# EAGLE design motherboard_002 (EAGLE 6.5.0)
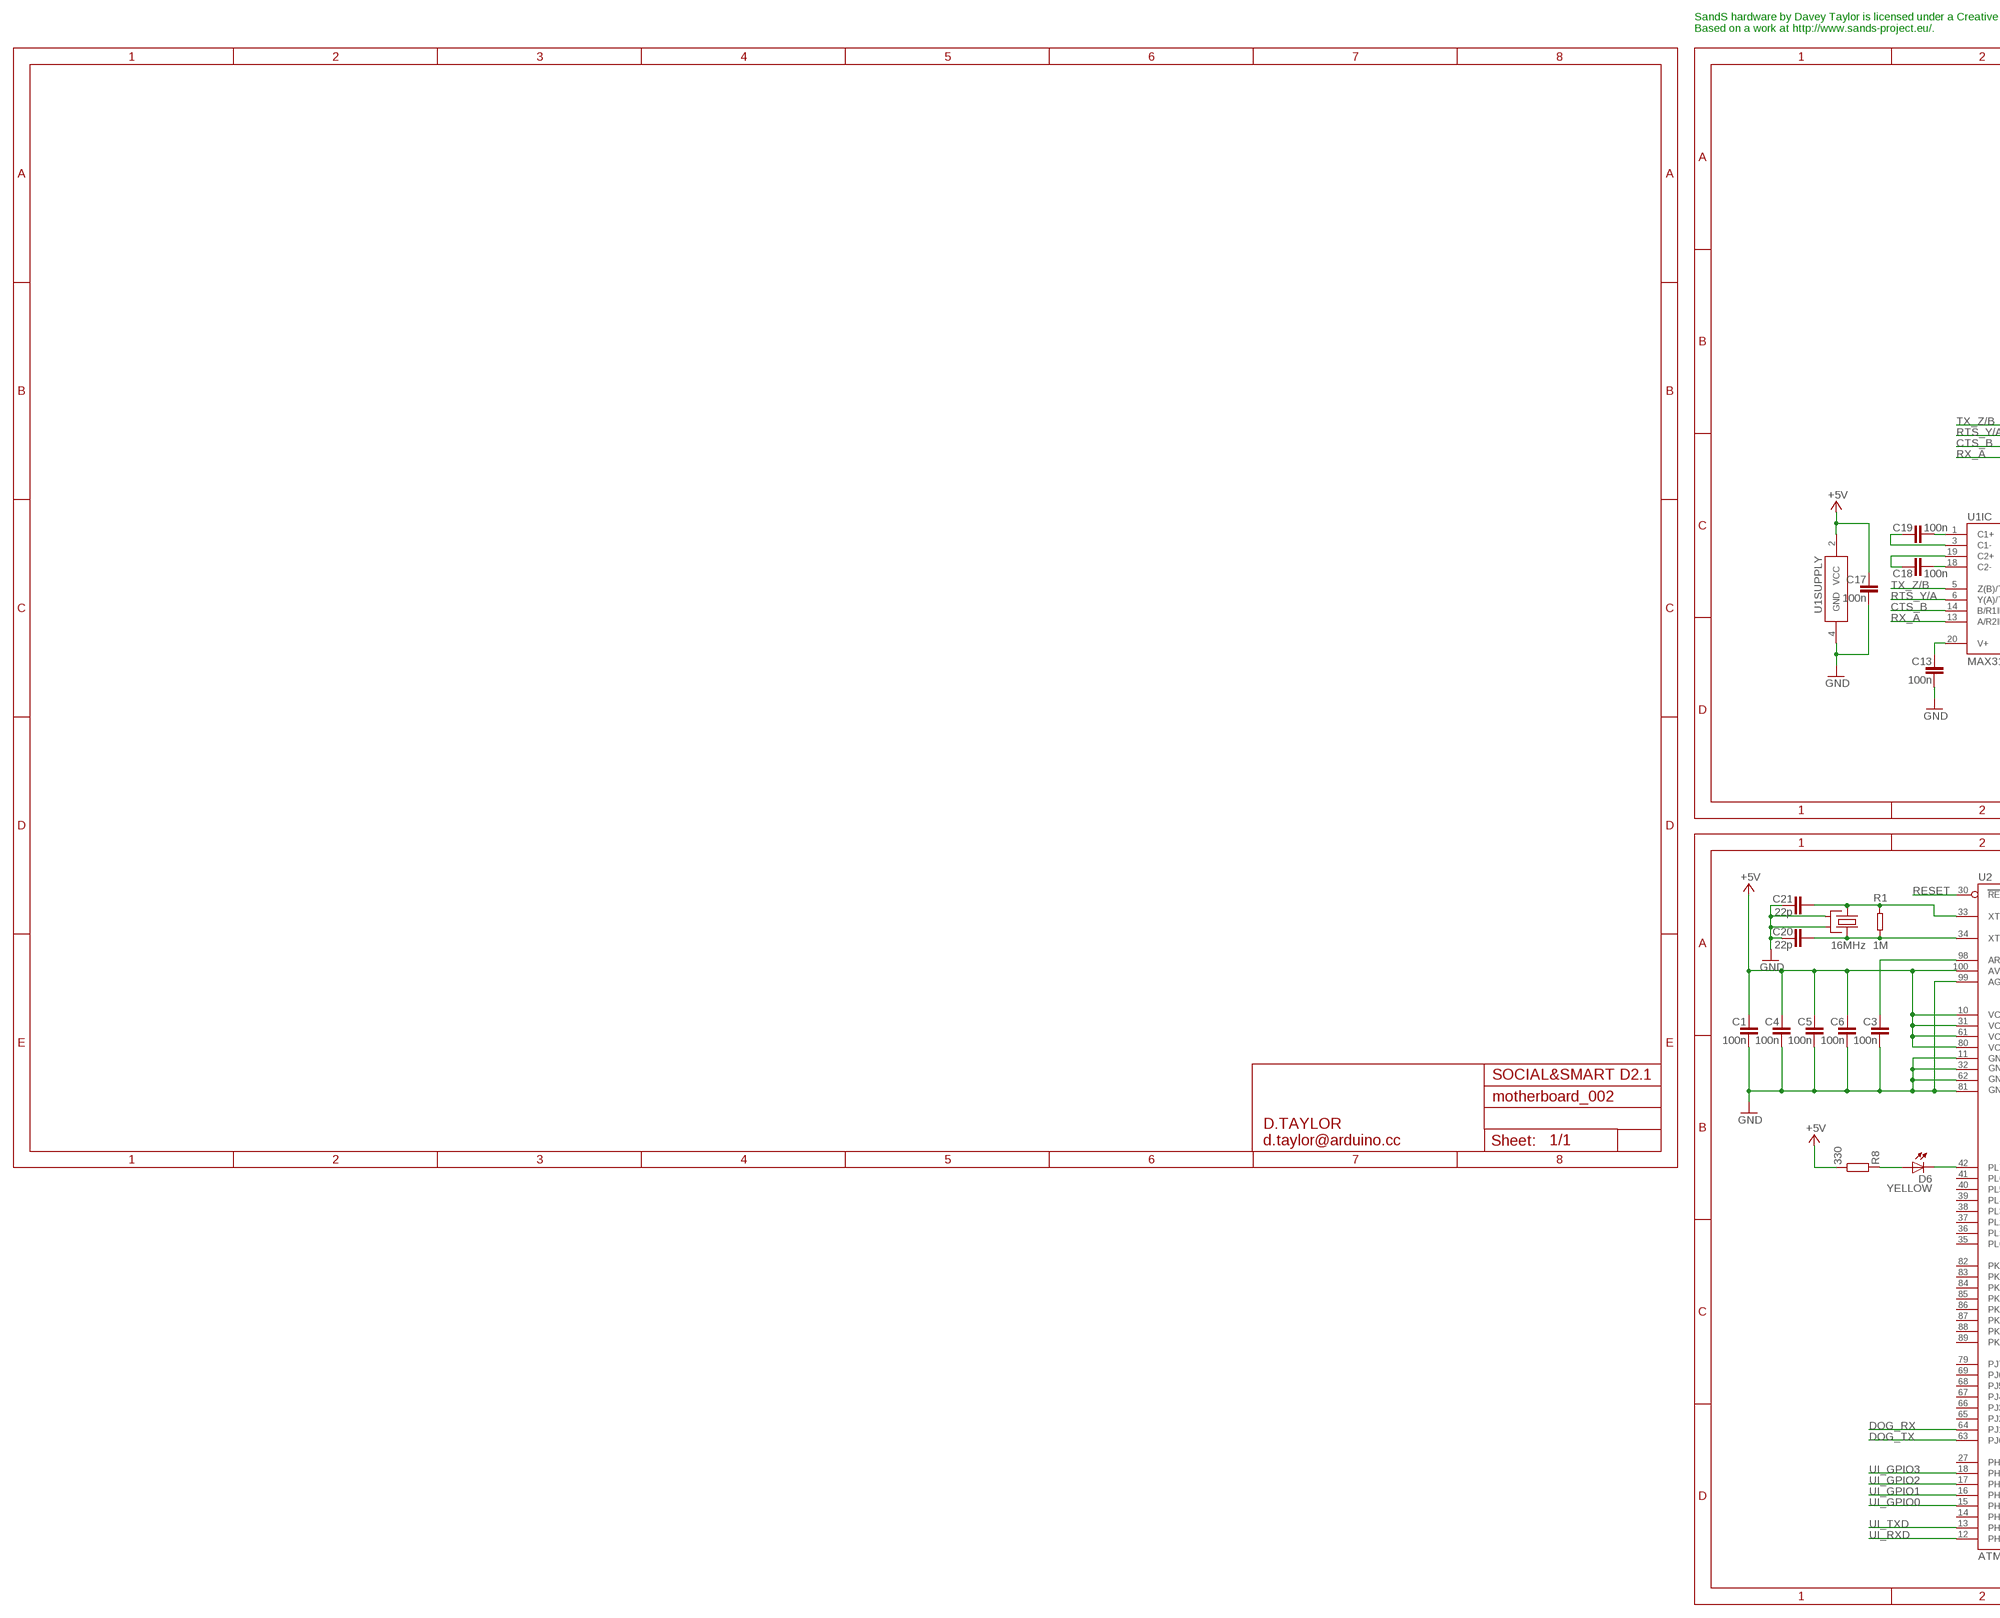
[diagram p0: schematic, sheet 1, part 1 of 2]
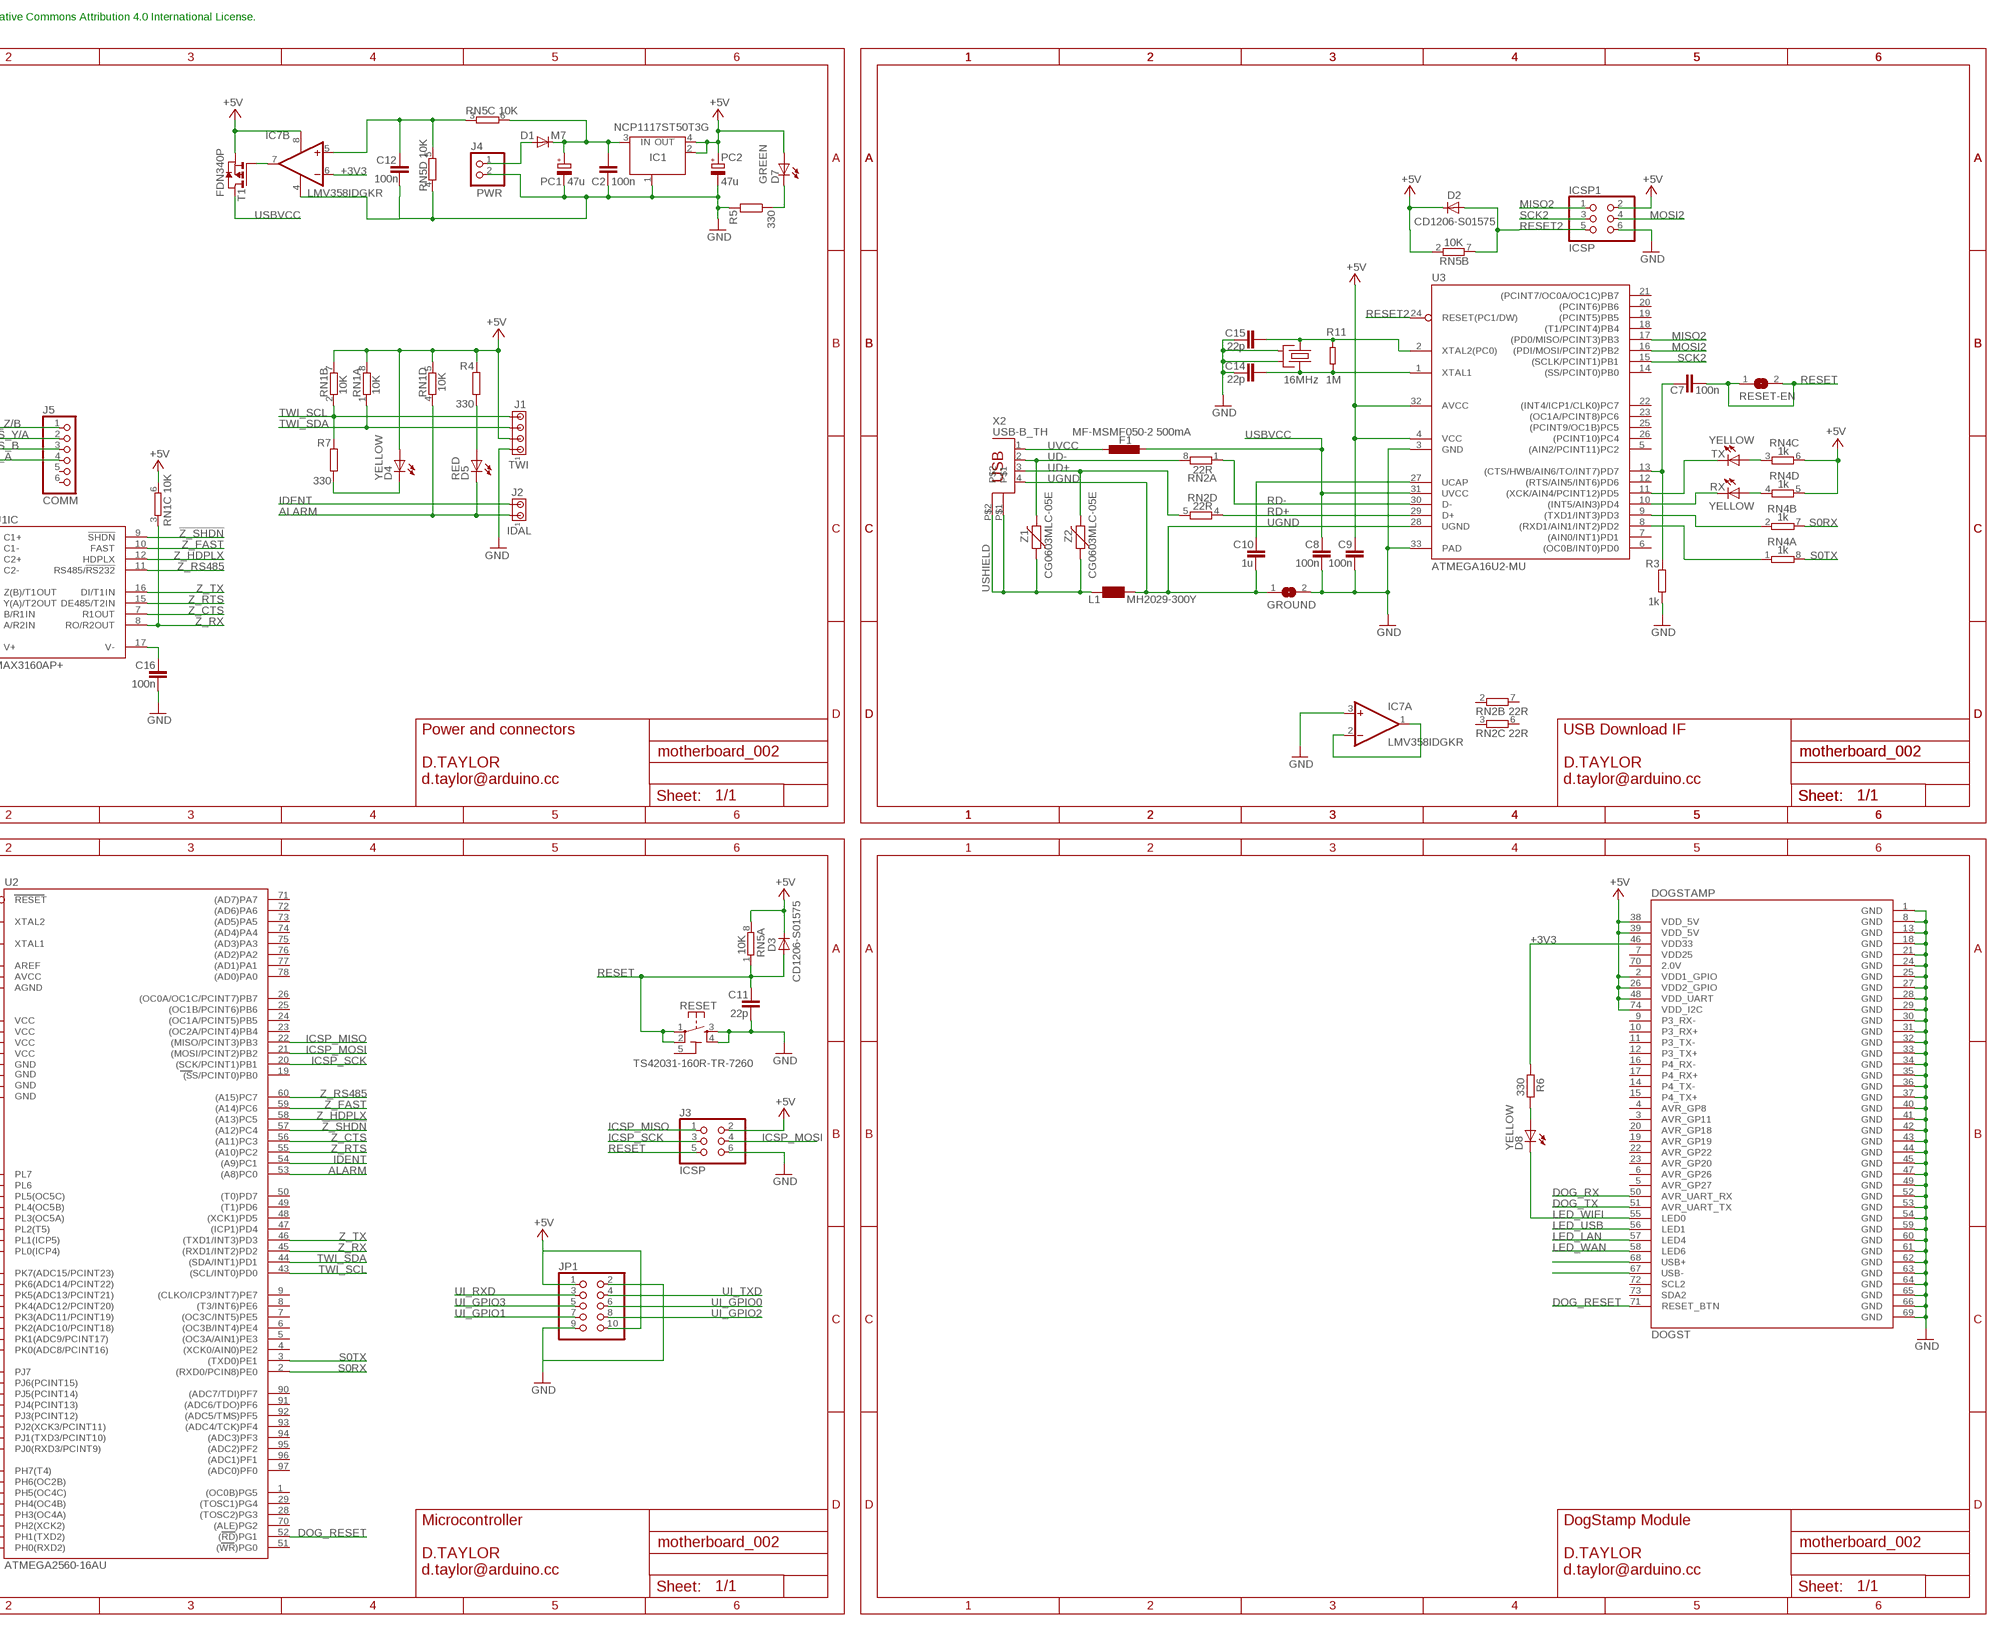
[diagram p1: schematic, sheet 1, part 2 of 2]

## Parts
C1  100n  C-EU0603-RND  [C0603-ROUND]
C2  100n  C-EU0603-RND  [C0603-ROUND]
C3  100n  C-EU0603-RND  [C0603-ROUND]
C4  100n  C-EU0603-RND  [C0603-ROUND]
C5  100n  C-EU0603-RND  [C0603-ROUND]
C6  100n  C-EU0603-RND  [C0603-ROUND]
C7  100n  C-EU0603-RND  [C0603-ROUND]
C8  100n  C-EU0603-RND  [C0603-ROUND]
C9  100n  C-EU0603-RND  [C0603-ROUND]
C10  1u  C-EU0603-RND  [C0603-ROUND]
C11  22p  C-EU0603-RND  [C0603-ROUND]
C12  100n  C-EU0603-RND  [C0603-ROUND]
C13  100n  C-EU0603-RND  [C0603-ROUND]
C14  22p  C-EU0603-RND  [C0603-ROUND]
C15  22p  C-EU0603-RND  [C0603-ROUND]
C16  100n  C-EU0603-RND  [C0603-ROUND]
C17  100n  C-EU0603-RND  [C0603-ROUND]
C18  100n  C-EU0603-RND  [C0603-ROUND]
C19  100n  C-EU0603-RND  [C0603-ROUND]
C20  22p  C-EU0603-RND  [C0603-ROUND]
C21  22p  C-EU0603-RND  [C0603-ROUND]
D1  M7  DIODE-SMB  [SMB]
D2  CD1206-S01575  DIODE-MINIMELF  [MINIMELF]
D3  CD1206-S01575  DIODE-MINIMELF  [MINIMELF]
D4  YELLOW  LEDCHIP-LED0805  [CHIP-LED0805]
D5  RED  LEDCHIP-LED0805  [CHIP-LED0805]
D6  YELLOW  LEDCHIP-LED0805  [CHIP-LED0805]
D7  GREEN  LEDCHIP-LED0805  [CHIP-LED0805]
D8  YELLOW  LEDCHIP-LED0805  [CHIP-LED0805]
DOGSTAMP  DOGST  [DOGST]
F1  MF-MSMF050-2 500mA  L-EUL1812  [L1812]
GROUND  SJ  [SJ]
IC1  NCP1117ST50T3G  MC33269ST-3.3T3  [SOT223]
IC7  LMV358IDGKR  LMV358MMX  [MSOP08]
ICSP1  ICSP  PINHD-2X3  [2X03]
J1  TWI  MTA04-100  [10X04MTA]
J2  IDAL  MTA02-100  [10X02MTA]
J3  ICSP  PINHD-2X3  [2X03]
J4  PWR  MKDS_1,5/2-5,08  [MKDS1,5/2-5,08]
J5  COMM  PINHD-1X6  [1X06]
JP1  PINHD-2X5  [2X05]
L1  MH2029-300Y  WE-CBF_0805  [0805]
PC1  47u  CPOL-EUD  [PANASONIC_D]
PC2  47u  CPOL-EUD  [PANASONIC_D]
R1  1M  R-EU_0603-RND  [R0603-ROUND]
R3  1k  R-EU_R0603  [R0603-ROUND]
R4  330  R-EU_R0603  [R0603-ROUND]
R5  330  R-EU_R0603  [R0603-ROUND]
R6  330  R-EU_R0603  [R0603-ROUND]
R7  330  R-EU_R0603  [R0603-ROUND]
R8  330  R-EU_R0603  [R0603-ROUND]
R11  1M  R-EU_0603-RND  [R0603-ROUND]
RESET  TS42031-160R-TR-7260  TS42  [TS42]
RESET-EN  SJ  [SJ]
RN1  10K  4R-NCAT16  [CAT16]
RN2  22R  4R-NCAY16  [CAY16]
RN4  1k  4R-NCAY16  [CAY16]
RN5  10K  4R-NCAT16  [CAT16]
RX  YELLOW  LEDCHIP-LED0805  [CHIP-LED0805]
T1  FDN340P  PMOSSOT23  [SOT-23]
TX  YELLOW  LEDCHIP-LED0805  [CHIP-LED0805]
U1  MAX3160AP+  [SSOP20]
U2  ATMEGA2560-16AU  ATMEGA25602560-16AU  [TQFP100]
U3  ATMEGA16U2-MU  [MLF32]
X1  16MHz  CRYSTAL2-KX7  [XTAL-3.2-2.5]
X2  USB-B_TH  PN61729  [PN61729]
X3  16MHz  CRYSTAL2-KX7  [XTAL-3.2-2.5]
Z1  CG0603MLC-05E  VARISTORCN0603  [CT/CN0603]
Z2  CG0603MLC-05E  VARISTORCN0603  [CT/CN0603]

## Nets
!Z_SHDN!: U1.9(IC:!SHDN!) U2.57((A12)PC4)
+3V3 [power]: DOGSTAMP.46(VDD33) IC7.6(B:-IN) R6.2
+5V: C1.1 C4.1 C5.1 C6.1 C9.1 C17.1 D2.C D3.C D4.A D7.A DOGSTAMP.2(VDD1_GPIO) DOGSTAMP.26(VDD2_GPIO) DOGSTAMP.38(VDD_5V) DOGSTAMP.39(VDD_5V) DOGSTAMP.48(VDD_UART) DOGSTAMP.74(VDD_I2C) IC1.2(OUT) IC1.4(OUT) IC7.8(P:V+) ICSP1.2 J1.2 J3.2 JP1.1 JP1.10 PC2.+ R4.2 R8.1 RN1.5 RN1.6 RN1.7 RN1.8 RN4.5 RN4.6 RN5.2 RN5.8 T1.2(S) U1.2(SUPPLY:VCC) U2.10(VCC) U2.31(VCC1) U2.61(VCC2) U2.80(VCC3) U2.100(AVCC) U3.4(VCC) U3.32(AVCC)
ALARM: D5.C J2.1 RN1.4 U2.53((A8)PC0)
CMP: C12.2 IC7.5(B:+IN) RN5.3 RN5.5
CTS_B: J5.3 U1.14(IC:B/R1IN)
DOG_RESET: DOGSTAMP.71(RESET_BTN) U2.52((RD)PG1)
DOG_RX: DOGSTAMP.50(AVR_UART_RX) U2.64(PJ1(TXD3/PCINT10))
DOG_TX: DOGSTAMP.51(AVR_UART_TX) U2.63(PJ0(RXD3/PCINT9))
DTR: C7.1 R3.2 U3.13((CTS/HWB/AIN6/TO/INT7)PD7)
GATE_CMD: IC7.7(B:OUT) T1.3(G)
GND: C1.2 C2.2 C3.2 C4.2 C5.2 C6.2 C8.2 C9.2 C11.2 C12.1 C13.2 C14.2 C15.2 C16.2 C17.2 C20.2 C21.2 DOGSTAMP.1(GND) DOGSTAMP.8(GND) DOGSTAMP.13(GND) DOGSTAMP.18(GND) DOGSTAMP.21(GND) DOGSTAMP.24(GND) DOGSTAMP.25(GND) DOGSTAMP.27(GND) DOGSTAMP.28(GND) DOGSTAMP.29(GND) DOGSTAMP.30(GND) DOGSTAMP.31(GND) DOGSTAMP.32(GND) DOGSTAMP.33(GND) DOGSTAMP.34(GND) DOGSTAMP.35(GND) DOGSTAMP.36(GND) DOGSTAMP.37(GND) DOGSTAMP.40(GND) DOGSTAMP.41(GND) DOGSTAMP.42(GND) DOGSTAMP.43(GND) DOGSTAMP.44(GND) DOGSTAMP.45(GND) DOGSTAMP.47(GND) DOGSTAMP.49(GND) DOGSTAMP.52(GND) DOGSTAMP.53(GND) DOGSTAMP.54(GND) DOGSTAMP.59(GND) DOGSTAMP.60(GND) DOGSTAMP.61(GND) DOGSTAMP.62(GND) DOGSTAMP.63(GND) DOGSTAMP.64(GND) DOGSTAMP.65(GND) DOGSTAMP.66(GND) DOGSTAMP.69(GND) GROUND.2 IC1.1(GND/ADJ) IC7.3(A:+IN) IC7.4(P:V-) ICSP1.6 J1.1 J3.6 J4.2 JP1.2 JP1.9 PC1.- PC2.- R3.1 R5.2 RESET.3 RESET.4 RN5.4 U1.4(SUPPLY:GND) U2.11(GND) U2.32(GND1) U2.62(GND2) U2.81(GND3) U2.99(AGND) U3.3(GND) U3.33(PAD) X1.2(SH1) X1.4(SH2) X3.2(SH1) X3.4(SH2)
ICSP_MISO: J3.1 U2.22((MISO/PCINT3)PB3)
ICSP_MOSI: J3.4 U2.21((MOSI/PCINT2)PB2)
ICSP_SCK: J3.3 U2.20((SCK/PCINT1)PB1)
IDENT: J2.2 U2.54((A9)PC1)
LED_LAN: DOGSTAMP.57(LED4)
LED_USB: DOGSTAMP.56(LED1)
LED_WAN: DOGSTAMP.58(LED6)
LED_WIFI: D8.C DOGSTAMP.55(LED0)
M8RXD: RN4.2 U3.9((TXD1/INT3)PD3)
M8TXD: RN4.1 U3.8((RXD1/AIN1/INT2)PD2)
MISO2: ICSP1.1 U3.17((PD0/MISO/PCINT3)PB3)
MOSI2: ICSP1.4 U3.16((PDI/MOSI/PCINT2)PB2)
N$1: C3.1 U2.98(AREF)
N$2: IC7.1(A:OUT) IC7.2(A:-IN)
N$3: C14.1 R11.1 U3.1(XTAL1) X1.3(X2)
N$4: DOGSTAMP.68(USB+)
N$5: D5.A R4.1
N$6: C19.2 U1.1(IC:C1+)
N$7: C18.2 U1.18(IC:C2-)
N$8: C18.1 U1.19(IC:C2+)
N$9: C19.1 U1.3(IC:C1-)
N$10: C13.1 U1.20(IC:V+)
N$11: C16.1 U1.17(IC:V-)
N$12: D7.C R5.1
N$13: D8.A R6.1
N$14: D4.C R7.1
N$15: D6.C U2.42(PL7)
N$16: D6.A R8.2
N$17: DOGSTAMP.67(USB-)
N$21: C20.1 R1.1 U2.34(XTAL1) X3.3(X2)
N$54: RN4.4 RX.A
N$55: RN4.3 TX.A
PWRIN [power]: D1.A J4.1
RD+: RN2.4 U3.29(D+)
RD-: RN2.1 U3.30(D-)
RESET: C7.2 C11.1 D3.A J3.5 RESET-EN.1 RESET-EN.2 RESET.1 RESET.2 RN5.1 U2.30(RESET)
RESET2: D2.A ICSP1.5 RN5.7 U3.24(RESET(PC1/DW))
RTS_Y/A: J5.2 U1.6(IC:Y(A)/T2OUT)
RX_A: J5.4 U1.13(IC:A/R2IN)
RXL: RX.C U3.10((INT5/AIN3)PD4)
S0RX: RN4.7 U2.2((RXD0/PCIN8)PE0)
S0TX: RN4.8 U2.3((TXD0)PE1)
SCK2: ICSP1.3 U3.15((SCLK/PCINT1)PB1)
TWI_SCL: J1.4 R7.2 RN1.2 U2.43((SCL/INT0)PD0)
TWI_SDA: J1.3 RN1.1 U2.44((SDA/INT1)PD1)
TX_Z/B: J5.1 U1.5(IC:Z(B)/T1OUT)
TXL: TX.C U3.11((XCK/AIN4/PCINT12)PD5)
UD+: RN2.5 X2.3 Z2.2
UD-: RN2.8 X2.2 Z1.2
UGND [gnd]: C10.2 GROUND.1 L1.1 U3.28(UGND) X2.4
UI_GPIO0: JP1.6 U2.15(PH3(OC4A))
UI_GPIO1: JP1.7 U2.16(PH4(OC4B))
UI_GPIO2: JP1.8 U2.17(PH5(OC4C))
UI_GPIO3: JP1.5 U2.18(PH6(OC2B))
UI_RXD: JP1.3 U2.12(PH0(RXD2))
UI_TXD: JP1.4 U2.13(PH1(TXD2))
USBVCC [power usb]: C8.1 F1.1 T1.1(D) U3.31(UVCC)
USHIELD [gnd]: L1.2 X2.P$1 X2.P$2 Z1.1 Z2.1
UVCC [power usb]: F1.2 X2.1
VIN [power]: C2.1 D1.C IC1.3(IN) PC1.+ RN5.6
VUCAP: C10.1 U3.27(UCAP)
XT1: C21.1 R1.2 U2.33(XTAL2) X3.1(X1)
XT2: C15.1 R11.2 U3.2(XTAL2(PC0)) X1.1(X1)
Z_CTS: U1.7(IC:R1OUT) U2.56((A11)PC3)
Z_FAST: U1.10(IC:FAST) U2.59((A14)PC6)
Z_HDPLX: U1.12(IC:HDPLX) U2.58((A13)PC5)
Z_RS485: U1.11(IC:RS485/!RS232!) U2.60((A15)PC7)
Z_RTS: U1.15(IC:DE485/T2IN) U2.55((A10)PC2)
Z_RX: RN1.3 U1.8(IC:RO/R2OUT) U2.45((RXD1/INT2)PD2)
Z_TX: U1.16(IC:DI/T1IN) U2.46((TXD1/INT3)PD3)
Unconnected: DOGSTAMP.3(AVR_GP11) DOGSTAMP.4(AVR_GP8) DOGSTAMP.5(AVR_GP27) DOGSTAMP.6(AVR_GP26) DOGSTAMP.7(VDD25) DOGSTAMP.9(P3_RX-) DOGSTAMP.10(P3_RX+) DOGSTAMP.11(P3_TX-) DOGSTAMP.12(P3_TX+) DOGSTAMP.14(P4_TX-) DOGSTAMP.15(P4_TX+) DOGSTAMP.16(P4_RX-) DOGSTAMP.17(P4_RX+) DOGSTAMP.19(AVR_GP19) DOGSTAMP.20(AVR_GP18) DOGSTAMP.22(AVR_GP22) DOGSTAMP.23(AVR_GP20) DOGSTAMP.70(2.0V) DOGSTAMP.72(SCL2) DOGSTAMP.73(SDA2) J5.5 J5.6 RN2.2 RN2.3 RN2.6 RN2.7 U2.1((OC0B)PG5) U2.4((XCK0/AIN0)PE2) U2.5((OC3A/AIN1)PE3) U2.6((OC3B/INT4)PE4) U2.7((OC3C/INT5)PE5) U2.8((T3/INT6)PE6) U2.9((CLKO/ICP3/INT7)PE7) U2.14(PH2(XCK2)) U2.19((SS/PCINT0)PB0) U2.23((OC2A/PCINT4)PB4) U2.24((OC1A/PCINT5)PB5) U2.25((OC1B/PCINT6)PB6) U2.26((OC0A/OC1C/PCINT7)PB7) U2.27(PH7(T4)) U2.28((TOSC2)PG3) U2.29((TOSC1)PG4) U2.35(PL0(ICP4)) U2.36(PL1(ICP5)) U2.37(PL2(T5)) U2.38(PL3(OC5A)) U2.39(PL4(OC5B)) U2.40(PL5(OC5C)) U2.41(PL6) U2.47((ICP1)PD4) U2.48((XCK1)PD5) U2.49((T1)PD6) U2.50((T0)PD7) U2.51((WR)PG0) U2.65(PJ2(XCK3/PCINT11)) U2.66(PJ3(PCINT12)) U2.67(PJ4(PCINT13)) U2.68(PJ5(PCINT14)) U2.69(PJ6(PCINT15)) U2.70((ALE)PG2) U2.71((AD7)PA7) U2.72((AD6)PA6) U2.73((AD5)PA5) U2.74((AD4)PA4) U2.75((AD3)PA3) U2.76((AD2)PA2) U2.77((AD1)PA1) U2.78((AD0)PA0) U2.79(PJ7) U2.82(PK7(ADC15/PCINT23)) U2.83(PK6(ADC14/PCINT22)) U2.84(PK5(ADC13/PCINT21)) U2.85(PK4(ADC12/PCINT20)) U2.86(PK3(ADC11/PCINT19)) U2.87(PK2(ADC10/PCINT18)) U2.88(PK1(ADC9/PCINT17)) U2.89(PK0(ADC8/PCINT16)) U2.90((ADC7/TDI)PF7) U2.91((ADC6/TDO)PF6) U2.92((ADC5/TMS)PF5) U2.93((ADC4/TCK)PF4) U2.94((ADC3)PF3) U2.95((ADC2)PF2) U2.96((ADC1)PF1) U2.97((ADC0)PF0) U3.5((AIN2/PCINT11)PC2) U3.6((OC0B/INT0)PD0) U3.7((AIN0/INT1)PD1) U3.12((RTS/AIN5/INT6)PD6) U3.14((SS/PCINT0)PB0) U3.18((T1/PCINT4)PB4) U3.19((PCINT5)PB5) U3.20((PCINT6)PB6) U3.21((PCINT7/OC0A/OC1C)PB7) U3.22((INT4/ICP1/CLK0)PC7) U3.23((OC1A/PCINT8)PC6) U3.25((PCINT9/OC1B)PC5) U3.26((PCINT10)PC4)

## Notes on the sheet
- SandS hardware by Davey Taylor is licensed under a Creative Commons Attribution 4.0 International License.
  Based on a work at http://www.sands-project.eu/.
- Power and connectors
  
  D.TAYLOR
  d.taylor@arduino.cc
- USB Download IF
  
  D.TAYLOR
  d.taylor@arduino.cc
- SOCIAL&SMART D2.1
- D.TAYLOR
  d.taylor@arduino.cc
- Microcontroller
  
  D.TAYLOR
  d.taylor@arduino.cc
- DogStamp Module
  
  D.TAYLOR
  d.taylor@arduino.cc

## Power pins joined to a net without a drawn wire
5-GND: RESET.5(5-GND)

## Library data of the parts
C1-C21 = SmartPrj:C-EU: CAPACITOR, European symbol
D1-D3 = diode:DIODE-: DIODE
D4-D8 RX TX = led:LED: LED
DOGSTAMP = d_taylor:DOGST
F1 = rcl:L-EU: INDUCTOR, European symbol
GROUND RESET-EN = jumper:SJ: SMD solder JUMPER
IC1 = linear:MC33269ST*: Adjustable Output Low Dropout Voltage Regulator 800 mA Source: http://www.onsemi.com/pub/Collateral/MC33269-D.PDF
IC7 = linear:LMV358?*: Dual General Purpose, Low Voltage, Rail-to-Rail Output Operational Amplifiers Source: http://www.national.com/mpf/LM/LMV321.html http://www.national.com/dt/lmv_qual.pdf
ICSP1 = SmartPrj:PINHD-2X3: PIN HEADER
J1 = con-amp:MTA04-100: AMP connector
J2 = con-amp:MTA02-100: AMP connector
J3 = pinhead:PINHD-2X3: PIN HEADER
J4 = d_taylor:MKDS_1,5/2-5,08: Screw terminal header
J5 = pinhead:PINHD-1X6: PIN HEADER
JP1 = pinhead:PINHD-2X5: PIN HEADER
L1 = wuerth-elektronik:WE-CBF: SMD EMI Suppression Ferrite Beads
PC1 PC2 = rcl:CPOL-EU: POLARIZED CAPACITOR, European symbol
R1 R11 = d_taylor:R-EU_: RESISTOR, European symbol
R3-R8 = SmartPrj:R-EU_: RESISTOR, European symbol
RESET = SmartPrj:TS42: TS42 Dongnan Electronics Tact switch VDC 12V - 50mA
RN1 RN2 RN4 RN5 = resistor-dil:4R-N: Array Chip Resistor Source: RS Component / Phycomp; OC_FARNELL: unknown; OC_NEWARK: unknown
T1 = zetex:PMOSSOT23: MOS FET; OC_FARNELL: unknown; OC_NEWARK: unknown
U1 = d_taylor:MAX3160*AP+
U2 = SmartPrj:ATMEGA2560: MICROCONTROLLER 64/128/256 Kbytes FLASH 4 Kbytes EEPROM 8 Kbytes SRAM 86 General Purpose I/O pins 12-channels16-bit PWM 4 x Serial USARTs 16-channels 10-bit A/D
U3 = SmartPrj:ATMEGA16U2-
X1 X3 = d_taylor:CRYSTAL2: KX7 SMD crystal
X2 = SmartPrj:PN61729: BERG USB connector
Z1 Z2 = varistor:VARISTOR: VARISTOR

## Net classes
0 default: width 0.203 mm, drill 0.406 mm, clearance 0.203 mm
1 power: width 0.61 mm, drill 0.406 mm, clearance 0.203 mm
2 gnd: width 0.305 mm, drill 0.406 mm, clearance 0.203 mm
3 power usb: width 0.508 mm, drill 0.406 mm, clearance 0.203 mm

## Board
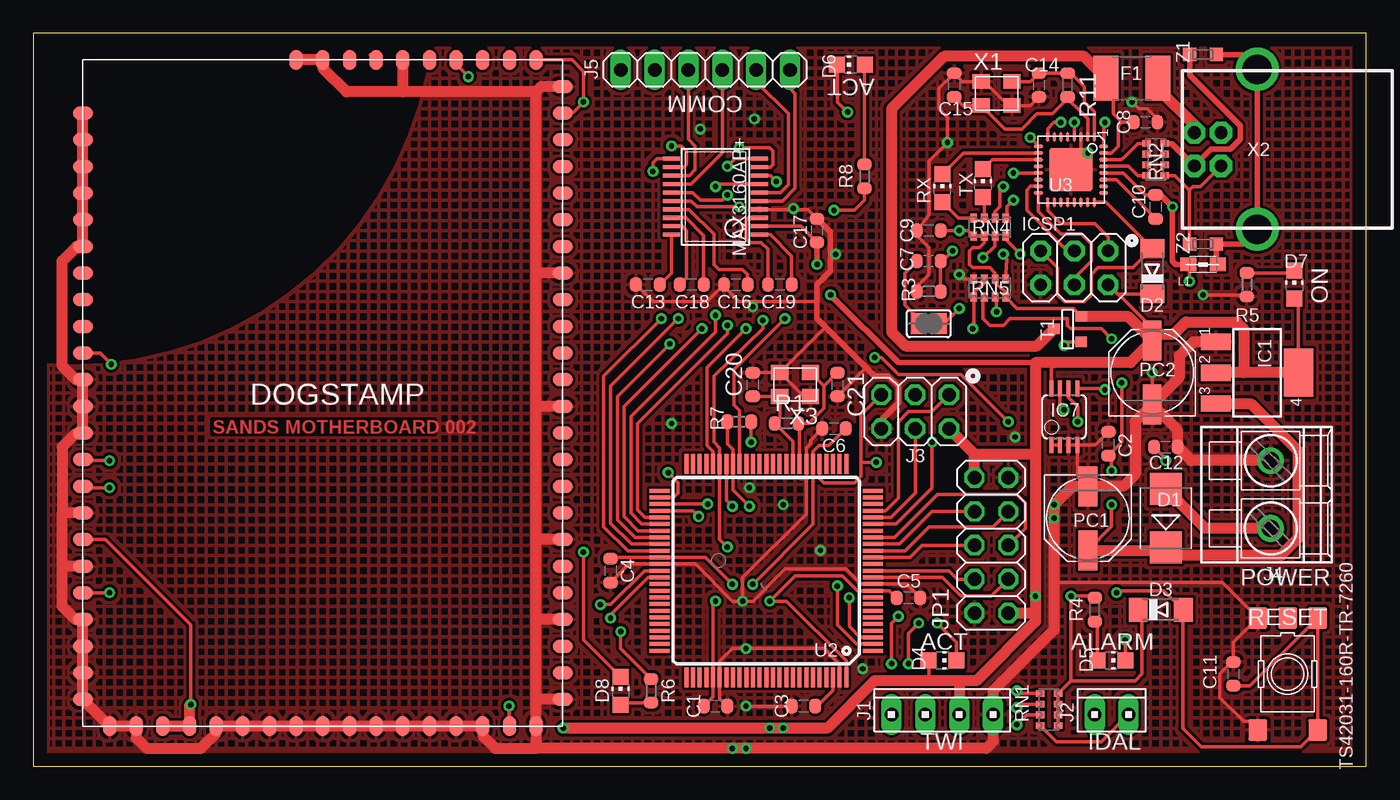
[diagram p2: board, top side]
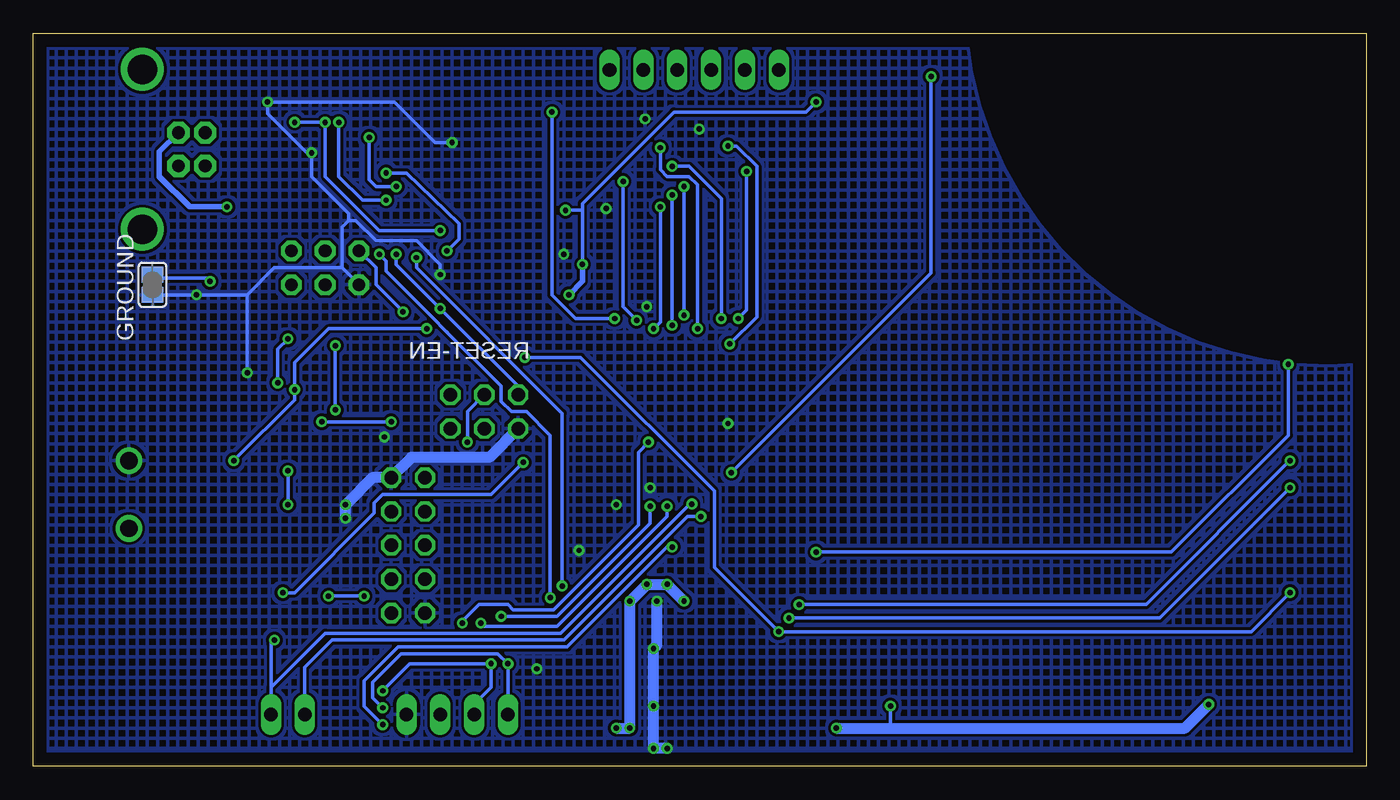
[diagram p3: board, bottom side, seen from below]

Size 100 x 55 mm. Coordinates in mm from the lower left corner, seen from the top.
Outline: 0,0 100,0 100,55 0,55 0,0
Copper layers (1*16): Top 0.035mm / dielectric 1.5mm / Bottom 0.035mm
Design rules "default *": minimum track width 10mil, minimum drill 16mil, track to track 8mil, track to pad 8mil, pad to pad 8mil, via to via 8mil, smd to smd 8mil, copper to edge 40mil, drill to drill 8mil, minimum pad ring 10mil, minimum via ring 8mil, stop-mask expansion 4mil, vias tented up to drill 0mil, thermal gap 10mil

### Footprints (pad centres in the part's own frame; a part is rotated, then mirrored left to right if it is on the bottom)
C0603-ROUND = smd 0.898 x 1.1: 1 -0.889,0; 2 0.889,0
SMB = smd 2.4 x 2.4: A 2.2,0; C -2.2,0
MINIMELF = smd 1.4 x 1.8: A 1.7,0; C -1.7,0
CHIP-LED0805 = smd 1.2 x 1.2: A 0,-1.05; C 0,1.05
DOGST = smd 1 x 1.5: 1 -23,18; 2 -21,18; 3 -19,18; 4 -17,18; 5 -15,18; 6 -13,18; 7 -11,18; 8 -9,18; 9 -7,18; 10 -5,18; 11 -3,18; 12 -1,18; 13 1,18; 14 3,18; 15 5,18; 16 7,18; 17 9,18; 18 11,18; 19 13,18; 20 15,18; 21 17,18; 22 19,18; 23 21,18; 24 23,18; 42 23,-18; 43 21,-18; 44 19,-18; 45 17,-18; 46 15,-18; 47 13,-18; 48 11,-18; 49 9,-18; 50 7,-18; 51 5,-18; 52 3,-18; 53 1,-18; 54 -1,-18; 55 -3,-18; 56 -5,-18; 57 -7,-18; 58 -9,-18; 59 -11,-18; 60 -13,-18; 61 -15,-18; 62 -17,-18; 63 -19,-18; 64 -21,-18 | smd 1.5 x 1: 25 25,16; 26 25,14; 27 25,12; 28 25,10; 29 25,8; 30 25,6; 31 25,4; 32 25,2; 33 25,0; 34 25,-2; 35 25,-4; 36 25,-6; 37 25,-8; 38 25,-10; 39 25,-12; 40 25,-14; 41 25,-16; 65 -25,-2; 66 -25,0; 67 -25,2; 68 -25,4; 69 -25,6; 70 -25,8; 71 -25,10; 72 -25,12; 73 -25,14; 74 -25,16
L1812 = smd 1.9 x 3.4: 1 -1.95,0; 2 1.95,0
SJ = smd 1.168 x 1.6: 1 -0.762,0; 2 0.762,0
SOT223 = smd 1.219 x 2.235: 1 -2.311,-3.099; 2 0,-3.099; 3 2.311,-3.099 | smd 3.6 x 2.2: 4 0,3.099
MSOP08 = smd 0.3 x 1.2: 1 -0.976,-2.113; 2 -0.326,-2.113; 3 0.324,-2.113; 4 0.974,-2.113; 5 0.974,2.112; 6 0.324,2.112; 7 -0.326,2.112; 8 -0.976,2.112
2X03 = drill 0.95 pad 1.55 octagon: 1 -2.54,-1.27; 2 -2.54,1.27; 3 0,-1.27; 4 0,1.27; 5 2.54,-1.27; 6 2.54,1.27
10X04MTA = drill 1.016 long: 1 3.81,0; 2 1.27,0; 3 -1.27,0; 4 -3.81,0
10X02MTA = drill 1.016 long: 1 1.27,0; 2 -1.27,0
2X03' = drill 1.016 octagon: 1 -2.54,-1.27; 2 -2.54,1.27; 3 0,-1.27; 4 0,1.27; 5 2.54,-1.27; 6 2.54,1.27
MKDS1,5/2-5,08 = drill 1.3 pad 2: 1 -2.54,0; 2 2.54,0
1X06 = drill 1.016 long: 1 -6.35,0; 2 -3.81,0; 3 -1.27,0; 4 1.27,0; 5 3.81,0; 6 6.35,0
2X05 = drill 1.016 octagon: 1 -5.08,-1.27; 2 -5.08,1.27; 3 -2.54,-1.27; 4 -2.54,1.27; 5 0,-1.27; 6 0,1.27; 7 2.54,-1.27; 8 2.54,1.27; 9 5.08,-1.27; 10 5.08,1.27
0805 = smd 1.2 x 1: 1 -1.1,0; 2 1.1,0
PANASONIC_D = smd 3 x 1.4: + 2.4,0; - -2.4,0
R0603-ROUND = smd 0.898 x 1.1: 1 -0.889,0; 2 0.889,0
TS42 = smd 1.6 x 1.4: 1 -4.2,2.25; 2 4.2,2.25; 3 -4.2,-2.25; 4 4.2,-2.25; 5 -4.2,0
CAT16 = smd 0.5 x 0.65: 1 -1.2,-0.675; 2 -0.4,-0.675; 3 0.4,-0.675; 4 1.2,-0.675; 5 1.2,0.675; 6 0.4,0.675; 7 -0.4,0.675; 8 -1.2,0.675
CAY16 = smd 0.5 x 0.65: 1 -1.2,-0.675; 2 -0.4,-0.675; 3 0.4,-0.675; 4 1.2,-0.675; 5 1.2,0.675; 6 0.4,0.675; 7 -0.4,0.675; 8 -1.2,0.675
SOT-23 = smd 0.787 x 0.889: 1 0.025,-1.016; 2 -0.94,1.016; 3 0.991,1.016
SSOP20 = smd 0.305 x 1.245: 1 -2.857,-3.302; 2 -2.222,-3.302; 3 -1.587,-3.302; 4 -0.952,-3.302; 5 -0.317,-3.302; 6 0.318,-3.302; 7 0.953,-3.302; 8 1.588,-3.302; 9 2.223,-3.302; 10 2.858,-3.302; 11 2.858,3.302; 12 2.223,3.302; 13 1.588,3.302; 14 0.953,3.302; 15 0.318,3.302; 16 -0.317,3.302; 17 -0.952,3.302; 18 -1.587,3.302; 19 -2.222,3.302; 20 -2.857,3.302
TQFP100 = smd 1.5 x 0.3: 1 -8,6; 2 -8,5.5; 3 -8,5; 4 -8,4.5; 5 -8,4; 6 -8,3.5; 7 -8,3; 8 -8,2.5; 9 -8,2; 10 -8,1.5; 11 -8,1; 12 -8,0.5; 13 -8,0; 14 -8,-0.5; 15 -8,-1; 16 -8,-1.5; 17 -8,-2; 18 -8,-2.5; 19 -8,-3; 20 -8,-3.5; 21 -8,-4; 22 -8,-4.5; 23 -8,-5; 24 -8,-5.5; 25 -8,-6; 51 8,-6; 52 8,-5.5; 53 8,-5; 54 8,-4.5; 55 8,-4; 56 8,-3.5; 57 8,-3; 58 8,-2.5; 59 8,-2; 60 8,-1.5; 61 8,-1; 62 8,-0.5; 63 8,0; 64 8,0.5; 65 8,1; 66 8,1.5; 67 8,2; 68 8,2.5; 69 8,3; 70 8,3.5; 71 8,4; 72 8,4.5; 73 8,5; 74 8,5.5; 75 8,6 | smd 0.3 x 1.5: 26 -6,-8; 27 -5.5,-8; 28 -5,-8; 29 -4.5,-8; 30 -4,-8; 31 -3.5,-8; 32 -3,-8; 33 -2.5,-8; 34 -2,-8; 35 -1.5,-8; 36 -1,-8; 37 -0.5,-8; 38 0,-8; 39 0.5,-8; 40 1,-8; 41 1.5,-8; 42 2,-8; 43 2.5,-8; 44 3,-8; 45 3.5,-8; 46 4,-8; 47 4.5,-8; 48 5,-8; 49 5.5,-8; 50 6,-8; 76 6,8; 77 5.5,8; 78 5,8; 79 4.5,8; 80 4,8; 81 3.5,8; 82 3,8; 83 2.5,8; 84 2,8; 85 1.5,8; 86 1,8; 87 0.5,8; 88 0,8; 89 -0.5,8; 90 -1,8; 91 -1.5,8; 92 -2,8; 93 -2.5,8; 94 -3,8; 95 -3.5,8; 96 -4,8; 97 -4.5,8; 98 -5,8; 99 -5.5,8; 100 -6,8
MLF32 = smd 0.7 x 0.28: 1 -2.45,1.75; 2 -2.45,1.25; 3 -2.45,0.75; 4 -2.45,0.25; 5 -2.45,-0.25; 6 -2.45,-0.75; 7 -2.45,-1.25; 8 -2.45,-1.75; 17 2.45,-1.75; 18 2.45,-1.25; 19 2.45,-0.75; 20 2.45,-0.25; 21 2.45,0.25; 22 2.45,0.75; 23 2.45,1.25; 24 2.45,1.75 | smd 0.28 x 0.7: 9 -1.75,-2.45; 10 -1.25,-2.45; 11 -0.75,-2.45; 12 -0.25,-2.45; 13 0.25,-2.45; 14 0.75,-2.45; 15 1.25,-2.45; 16 1.75,-2.45; 25 1.75,2.45; 26 1.25,2.45; 27 0.75,2.45; 28 0.25,2.45; 29 -0.25,2.45; 30 -0.75,2.45; 31 -1.25,2.45; 32 -1.75,2.45 | smd 3.254 x 3.254: 33 0,0
XTAL-3.2-2.5 = smd 1.3 x 1.1: 1 -1.15,-0.9; 2 1.15,-0.9; 3 1.15,0.9; 4 -1.15,0.9
PN61729 = drill 0.95 pad 1.676 octagon: 1 1.25,4.71; 2 -1.25,4.71; 3 -1.25,2.71; 4 1.25,2.71 | drill 2.2: P$1 -6,0; P$2 6,0
CT/CN0603 = smd 1 x 1: 1 -1,0; 2 1,0

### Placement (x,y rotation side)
C1  51.18,4.51 0 top
C2  80.64,24.2 90 top
C3  57.78,4.51 180 top
C4  43.31,14.67 270 top
C5  65.66,12.64 0 top
C6  60.07,25.34 180 top
C7  67.18,37.91 180 top
C8  83.44,48.33 0 top
C9  67.18,40.2 180 top
C10  84.2,41.98 90 top
C11  90.04,6.92 90 top
C12  84.96,23.94 180 top
C13  46.1,36.13 180 top
C14  75.44,51.12 270 top
C15  69.09,51.12 90 top
C16  52.7,36.13 180 top
C17  58.8,40.2 90 top
C18  49.4,36.13 0 top
C19  56.01,36.13 0 top
C20  53.98,28.64 90 top
C21  60.33,28.64 270 top
D1  84.96,18.61 90 top
D2  83.95,37.15 90 top
D3  84.58,11.75 0 top
D4  68.2,7.94 270 top
D5  80.9,7.94 270 top
D6  61.34,52.64 90 top
D7  94.61,36.13 0 top
D8  44.07,5.65 0 top
DOGSTAMP  21.72,28.01 270 top
F1  82.42,51.63 0 top
GROUND  91.06,36.13 270 bottom
IC1  91.82,29.53 270 top
IC7  77.34,26.23 0 top
ICSP1  78.11,37.4 180 top
J1  68.2,3.88 0 top
J2  80.9,3.88 0 top
J3  ICSP  [2X03']  66.17,26.61 180 top
J4  92.84,20.39 90 top
J5  50.42,52.26 180 top
JP1  71.88,16.58 90 top
L1  87.76,37.66 0 top
PC1  79.12,18.61 270 top
PC2  83.95,29.53 90 top
R1  56.52,25.72 0 top
R3  67.18,35.63 0 top
R4  79.63,11.75 90 top
R5  91.06,36.13 270 top
R6  46.35,5.65 90 top
R7  52.96,25.85 180 top
R8  62.36,44.26 90 top
R11  77.6,51.12 270 top
RESET  94.11,6.92 270 top
RESET-EN  67.18,33.21 0 top
RN1  76.2,4.26 270 top
RN2  84.2,45.53 270 top
RN4  71.75,40.45 180 top
RN5  71.75,35.88 180 top
RX  68.2,43.37 0 top
T1  77.6,32.83 270 top
TX  71.25,43.75 0 top
U1  51.18,42.74 90 top
U2  54.99,14.67 180 top
U3  77.85,44.77 270 top
X1  72.26,50.48 0 top
X2  91.82,46.29 90 top
X3  57.15,28.64 180 top
Z1  87.76,53.41 180 top
Z2  87.76,39.18 180 top

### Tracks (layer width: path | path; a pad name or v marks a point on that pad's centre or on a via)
!Z_SHDN!  (via drill 0.41)
  Top 0.254: v50.16,32.83 44.32,26.99 44.32,18.73 45.39,17.67 U2.57 | U1.9 55.31,44.96 55.5,45.15 55.5,46.17 55.24,46.42 v52.96,46.42
  Bottom 0.254: v52.96,46.42 52.96,44.77 52.45,44.26 50.8,44.26 50.16,43.63 v50.16,32.83
+3V3  (via drill 0.41)
  Top 0.254: DOGSTAMP.46 5.7,13.01 v5.71,13.02 | v78.36,25.85 78.36,26.99 77.67,27.68 IC7.6 | R6.2 44.07,8.83 v44.07,10.1 | v63.12,30.67 63.63,30.67 64.9,29.4 69.6,29.4 v73.15,25.85
  Bottom 0.254: v5.71,13.02 8.64,10.1 v44.07,10.1 48.9,14.92 48.9,20.64 58.93,30.67 v63.12,30.67 | v73.15,25.85 v78.36,25.85
+5V  (via drill 0.41)
  Top 0.254: v78.11,48.33 U3.4 | U3.32 80.3,48.49 v80.39,48.33 | C9.1 v69.47,40.2 70.13,40.2 RN4.5 RN4.6 71.36,39.29 70.99,38.93 70.48,38.93 70.23,38.67 70.23,37.66 70.48,37.4 71.75,37.4 72.16,37 RN5.2 72.16,36.24 72.14,36.26 72.95,35.57 RN5.8 | PC2.+ 84.45,32.44 ICSP1.2 81.33,35.45 D2.C | RN5.8 72.85,35.06 | IC7.8 76.37,30.08 76.58,30.29 | T1.2 78.03,34.36 73.8,34.36 RN5.8 | 76.88,5.44 RN1.7 RN1.6 RN1.5 | C17.1 57.59,40.52 U1.2 | RN1.8 76.88,5.44 | 76.88,5.44 77.85,6.42 | 77.85,6.42 82.68,6.42 83.19,6.92 83.19,11.37 83.06,11.5 D3.C | 77.85,6.42 v77.85,12.77 79.5,12.77 R4.2 | v51.18,12.38 50.99,12.2 U2.80 50.99,5.21 C1.1 | v52.45,13.66 50.44,15.67 U2.61 43.7,15.67 C4.1 | v53.98,13.66 58.49,18.17 U2.31 58.49,23.63 58.93,24.07 59.69,24.07 C6.1 | U2.100 60.99,7.91 56.52,12.38 v55.24,12.38 57.15,14.29 60.71,14.29 61.83,13.17 U2.10 64.24,13.17 C5.1 | DOGSTAMP.74 40.41,53.01 41.27,52.14 v41.27,49.85 40.51,49.09 39.8,49.09 DOGSTAMP.2 | D7.A 94.92,34.78 IC1.4 | D4.A 67.18,7.91 67.18,6.42 | R8.1 62.36,42.48 61.59,41.72 v60.07,41.72 | DOGSTAMP.26 35.69,3.37 v35.69,4.51 | DOGSTAMP.48 5.41,17.01 11.81,10.61 v11.81,4.64
  Top 0.406: 75.18,30.29 64.9,30.29 v59.82,35.37 | v58.8,37.66 C17.1
  Top 0.813: IC1.4 90.81,29.53 | 90.81,29.53 IC1.2 | 84.45,32.44 85.58,32.44 86.49,33.34 90.3,33.34 90.81,32.83 90.81,29.53 | T1.2 82.11,33.77 PC2.+ 82.31,30.29 76.58,30.29 75.18,30.29 75.18,23.43 | 75.18,23.43 v75.18,12.77 75.18,11.62 | 75.18,11.62 75.18,10.86 70.74,6.42 69.47,6.42 | 69.47,6.42 J1.2 69.47,3.37 | 69.47,6.42 67.18,6.42 63.12,6.42 59.56,2.86 v56.26,2.86 v55.24,2.86 v39.75,2.86 | v11.81,4.64 11.72,4.54 DOGSTAMP.38 DOGSTAMP.39 | JP1.10 70.61,23.43 | 70.61,23.43 J3.2 | 70.61,23.43 75.18,23.43 | JP1.1 74.93,11.5 75.18,11.62
  Bottom 0.254: v80.39,48.33 v78.11,48.33 78.11,44.26 74.04,40.2 v69.47,40.2 | v75.18,12.77 v77.85,12.77 | v58.8,37.66 58.8,41.72 | 58.8,41.72 58.8,42.23 51.94,49.09 42.04,49.09 v41.27,49.85 | v60.07,41.72 58.8,41.72 | v35.69,4.51 35.69,2.86
  Bottom 0.406: v59.82,35.37 58.8,36.39 v58.8,37.66
  Bottom 0.813: v39.75,2.86 35.69,2.86 13.59,2.86 v11.81,4.64 | v56.26,2.86 v55.24,2.86 v55.24,12.38 v53.98,13.66 v52.45,13.66 v51.18,12.38
ALARM  (via drill 0.41)
  Top 0.254: v50.59,19.67 U2.53 | RN1.4 76.74,1.84 79.63,1.84 80.14,1.84 J2.1 | D5.C 81.92,7.97 v81.92,9.46
  Bottom 0.254: J2.1 82.17,5.91 | 82.17,5.91 78.11,9.97 70.74,9.97 60.45,9.97 50.8,19.62 v50.59,19.67 | v81.92,9.46 82.17,9.21 82.17,5.91
CMP  (via drill 0.41)
  Top 0.254: C12.2 84.96,23.05 v84.96,22.93 | v80.39,28.26 80.31,28.34 IC7.5 | RN5.3 71.36,36.24 71.37,36.26 70.56,35.57 RN5.5 70.56,32.76 v70.48,32.83
  Bottom 0.254: v84.96,22.93 80.39,27.5 v80.39,28.26 80.39,30.29 77.85,32.83 v70.48,32.83
CTS_B
  Top 0.254: J5.3 51.69,46.04 49.34,43.69 U1.14
DOG_RESET  (via drill 0.41)
  Top 0.254: U2.52 48.05,20.17 48.39,20.51 48.39,21.27 v47.62,22.04 | v32.64,51.75 32,52.39 31.75,52.78 DOGSTAMP.71
  Bottom 0.254: v47.62,22.04 32.64,37.02 v32.64,51.75
DOG_RX  (via drill 0.41)
  Top 0.254: U2.64 46.11,14.17 43.31,11.37 v43.31,11.11 | v5.71,20.89 3.83,20.89 DOGSTAMP.50
  Bottom 0.254: v43.31,11.11 15.49,11.11 v5.71,20.89
DOG_TX  (via drill 0.41)
  Top 0.254: U2.63 45.85,14.67 43.31,12.13 v42.55,12.13 | v5.71,22.93 3.8,22.93 DOGSTAMP.51
  Bottom 0.254: v42.55,12.13 16.51,12.13 v5.71,22.93
DTR  (via drill 0.41)
  Top 0.254: U3.13 v73.54,44.52 v73.53,44.52 | v68.96,38.67 68.2,37.91 C7.1 R3.2
  Bottom 0.254: v73.53,44.52 72.77,44.52 72.01,44.52 68.07,40.71 68.07,39.56 v68.96,38.67
GATE_CMD  (via drill 0.41)
  Top 0.254: v77.34,31.56 77.62,31.84 T1.3 | IC7.7 77.02,27.06 v77.34,26.74
  Bottom 0.254: v77.34,26.74 v77.34,31.56
GND  (via drill 0.41)
  Top 0.254: U3.3 78.6,45.52 U3.33 78.61,44.77 v79.12,46.04 | C8.2 84.33,48.58 83.57,49.34 82.93,49.34 v82.42,49.85 | IC1.1 89.51,31.84 89.53,31.82 | v83.95,29.53 PC2.- | IC7.4 79.67,24.12 C2.2 | IC7.4 78.32,21.81 PC1.- | IC7.3 IC7.4 | R3.1 66.29,36.01 67.18,36.9 67.18,38.93 66.29,39.82 C9.2 67.18,41.34 67.18,45.41 v68.58,46.8 68.58,48.71 67.94,49.34 67.94,50.87 C15.2 69.71,51.39 X1.4 71.36,51.39 73.16,49.58 X1.2 | 58.61,41.28 C17.2 58.1,41.79 U1.4 | C13.2 46.48,34.86 50.55,34.86 C16.2 51.82,36.01 52.96,34.86 58.8,34.86 | RESET.4 91.21,3.37 90.81,3.37 89.03,5.15 89.03,6.92 89.92,7.81 C11.2 90.04,9.31 RESET.3 89.2,13.78 76.58,13.78 | C3.2 v53.47,4.51 | v53.21,12.38 53.98,12.38 56.39,14.8 60.96,14.8 62.09,13.67 65.52,13.67 C5.2 | v53.21,12.38 53.21,14.16 57.99,18.94 U2.32 57.99,23.89 58.29,24.2 58.29,24.45 C6.2 | v53.21,12.38 52.45,12.38 49.66,15.17 U2.62 44.7,15.17 C4.2 | U2.99 60.49,7.65 59.31,8.83 v53.47,8.83 52.45,8.83 51.49,7.87 U2.81 51.49,5.09 C1.2 | R5.2 90.93,35.37 v87.76,35.37 | RN5.4 69.81,36.55 v69.47,36.9 | 73.42,49.6 X1.2 | C14.2 74.79,49.58 X1.2 | C21.2 62.48,29.91 | X3.4 57.8,27.74 X3.2 | C20.2 55.99,29.53 X3.2 | X3.2 56.02,29.54 59.44,32.96
  Top 0.406: C17.2 59.82,40.07 59.82,37.15 58.8,36.13 58.8,34.86 58.8,33.59 59.44,32.96 62.48,29.91 63.12,29.28 64.14,29.28 64.9,28.51 64.9,27.24 63.63,25.97 J3.6
  Top 0.813: J4.2 86.87,22.93 C12.1 85.85,25.23 PC2.- | IC1.1 87.02,31.84 85.98,30.8 85.98,29.16 PC2.- | PC2.- 82.68,25.86 82.68,21.91 81.78,21.01 PC1.- 77.97,21.01 v76.58,19.62 v76.58,18.61 76.58,13.78 76.58,10.23 72.01,5.65 J1.1 72.01,1.84 71.5,1.34 v53.47,1.34 v52.45,1.34 37.72,1.34 | 2.16,15.01 2.16,19.01 | DOGSTAMP.64 DOGSTAMP.63 DOGSTAMP.62 DOGSTAMP.61 DOGSTAMP.60 DOGSTAMP.59 3.25,39.01 2.16,37.91 2.16,30.04 3.19,29.01 DOGSTAMP.54 DOGSTAMP.53 DOGSTAMP.52 3.67,24.96 3.17,24.96 2.16,23.94 2.16,19.01 | DOGSTAMP.49 2.16,19.01 | DOGSTAMP.47 2.16,15.01 | DOGSTAMP.41 | 37.72,1.34 DOGSTAMP.25 37.72,5.01 | 37.72,5.01 37.72,11.01 | 37.72,11.01 37.72,17.01 | 37.72,17.01 37.72,27.01 | 37.72,27.01 37.72,37.01 | 37.72,37.01 37.72,50.61 | 37.72,50.61 27.72,50.61 | 27.72,50.61 23.5,50.61 21.72,52.39 DOGSTAMP.66 DOGSTAMP.65 | DOGSTAMP.69 27.72,50.61 | DOGSTAMP.1 38.1,51.01 37.72,50.61 | DOGSTAMP.8 37.72,37.01 | DOGSTAMP.18 37.72,17.01 | DOGSTAMP.13 37.72,27.01 | DOGSTAMP.24 37.72,5.01 | DOGSTAMP.21 37.72,11.01 | 37.72,1.34 34.67,1.34 33.72,2.29 DOGSTAMP.27 DOGSTAMP.28 DOGSTAMP.29 DOGSTAMP.30 DOGSTAMP.31 DOGSTAMP.32 DOGSTAMP.33 DOGSTAMP.34 DOGSTAMP.35 DOGSTAMP.36 DOGSTAMP.37 13.72,2.48 12.57,1.34 8.51,1.34 7.72,2.13 DOGSTAMP.40 DOGSTAMP.41 | DOGSTAMP.41 DOGSTAMP.42 DOGSTAMP.43 DOGSTAMP.44 DOGSTAMP.45 3.16,11.01 2.16,12 2.16,15.01
  Bottom 0.254: ICSP1.6 76.83,37.4 | 76.83,37.4 76.83,40.45 76.33,40.96 | GROUND.2 v87.76,35.37 83.95,35.37 | 83.95,35.37 81.92,37.4 76.83,37.4 | 83.95,35.37 v83.95,29.53 | v69.47,36.9 69.47,37.66 71.25,39.44 74.3,39.44 75.82,40.96 76.33,40.96 | 76.33,40.96 76.33,41.47 79.12,44.26 v79.12,46.04 79.5,46.04 82.42,48.96 v82.42,49.85 72.9,49.85 69.85,46.8 v68.58,46.8
  Bottom 0.813: v52.45,1.34 v53.47,1.34 v53.47,4.51 v53.47,8.83 53.21,9.08 v53.21,12.38 | v76.58,18.61 v76.58,19.62 74.55,21.66 JP1.9 71.63,23.18 65.79,23.18 J3.6
  other vias: 47.88,25.72 59.05,16.2 56.26,19.62 53.72,20.89 50.04,47.82 60.2,38.42 73.66,24.7 62.23,7.3 54.1,48.58 53.98,34.48 57.02,41.85
  pour Bottom (hatched): 0.13,30.16 0.13,0.19 99.95,0.19 99.95,54.55 29.97,54.55 arc-90 0.25,30.16
  pour Top (hatched): 0.13,30.16 0.13,0.19 99.95,0.19 99.95,54.55 29.97,54.55 arc-90 0.25,30.16
ICSP_MISO
  Top 0.254: U2.22 63.94,19.17 64.9,20.13 64.9,25.85 65.66,26.61 67.44,26.61 J3.1
ICSP_MOSI
  Top 0.254: U2.21 64.33,18.67 66.17,20.51 J3.4
ICSP_SCK  (via drill 0.41)
  Top 0.254: U2.20 64.71,18.17 67.44,20.89 v67.44,24.32
  Bottom 0.254: v67.44,24.32 67.44,26.61 J3.3
IDENT  (via drill 0.41)
  Top 0.254: v49.91,18.73 49.48,19.17 U2.54
  Bottom 0.254: J2.2 79.63,7.43 77.6,9.46 70.48,9.46 60.2,9.46 50.93,18.73 v49.91,18.73
LED_WIFI  (via drill 0.41)
  Top 0.254: D8.C 41.27,9.5 v41.27,16.07 | v5.84,30.16 5,31.01 DOGSTAMP.55
  Bottom 0.254: v41.27,16.07 14.61,16.07 5.84,24.83 v5.84,30.16
M8RXD  (via drill 0.41)
  Top 0.254: U3.9 75.4,46.58 v74.8,47.18 | v72.77,43.5 72.52,43.25 72.52,41.98 72.16,41.61 RN4.2
  Bottom 0.254: v74.8,47.18 74.8,44.01 74.3,43.5 v72.77,43.5
M8TXD  (via drill 0.41)
  Top 0.254: RN4.1 73.04,41.21 73.04,41.99 v73.53,42.48 | U3.8 76.1,47.85 76.58,48.33 v77.09,48.33
  Bottom 0.254: v77.09,48.33 77.09,44.26 75.31,42.48 v73.53,42.48
MISO2
  Top 0.254: U3.17 76.1,41.69 77.09,40.71 79.63,40.71 80.64,39.69 ICSP1.1
MOSI2
  Top 0.254: U3.16 75.4,41.63 77.09,39.94 78.61,39.94 79.38,39.18 79.38,37.91 78.11,36.64 ICSP1.4
N$1
  Top 0.254: C3.1 58.8,4.51 59.99,5.7 U2.98
N$2
  Top 0.254: IC7.2 IC7.1
N$3
  Top 0.254: U3.1 79.6,49.12 78.87,49.85 78.87,50.23 78.87,50.99 77.85,52.01 R11.1 C14.1 74.81,51.39 X1.3 73.42,51.37
N$4
  Top 0.254: 25.27,53.41 25.44,53.41 DOGSTAMP.68
N$5
  Top 0.254: R4.1 79.85,10.64 D5.A
N$6
  Top 0.254: U1.1 55.31,39.88 56.9,38.29 C19.2
N$7
  Top 0.254: U1.18 48.96,41.15 50.29,39.82 C18.2
N$8
  Top 0.254: U1.19 48.7,40.52 49.02,40.2 49.02,36.64 C18.1
N$9
  Top 0.254: U1.3 53.66,41.15 53.47,40.96 53.47,39.56 53.72,39.31 54.61,39.31 55.12,38.8 C19.1
N$10
  Top 0.254: U1.20 47.88,37.02 C13.1
N$11
  Top 0.254: U1.17 49.21,41.79 51.05,39.94 51.05,37.66 51.44,37.28 53.21,37.28 53.59,36.9 C16.1
N$12
  Top 0.254: D7.C 94.45,37.02 R5.1
N$13
  Top 0.254: D8.A 44.23,4.77 R6.1
N$14  (via drill 0.41)
  Top 0.254: D4.C 69.25,7.97 69.25,9.3 v67.82,10.73 | v53.85,24.32 R7.1
  Bottom 0.254: v67.82,10.73 67.82,10.86 66.55,12.13 64.39,12.13 64.01,11.75 60.96,11.75 54.61,18.1 54.61,19.5 54.61,23.56 v53.85,24.32
N$15  (via drill 0.41)
  Top 0.254: v56.39,33.59 52.58,29.78 52.58,27.12 52.99,26.7 U2.42 | v61.09,49.09 60.33,49.85 60.33,52.52 D6.C
  Bottom 0.254: v56.39,33.59 59.31,33.59 61.09,35.37 v61.09,49.09
N$16
  Top 0.254: D6.A 62.39,52.3 62.36,52.14 R8.2
N$21
  Top 0.254: U2.34 56.99,24.35 R1.1 56,26.09 X3.3 C20.1
N$54
  Top 0.254: RX.A 69.39,41.13 RN4.4
N$55
  Top 0.254: RN4.3 71.36,43.07 TX.A
PWRIN
  Top 0.813: J4.1 87.92,17.85 D1.A
RD+
  Top 0.254: RN2.4 82.86,44.33 82.42,44.77 82.17,45.02 U3.29
RD-
  Top 0.254: RN2.1 82.86,46.73 81.92,45.79 81.65,45.52 U3.30
RESET  (via drill 0.41)
  Top 0.254: RN5.1 72.95,36.97 73.03,38.04 v72.77,38.42 | C7.2 65.41,37.02 65.41,34.61 66.42,33.59 RESET-EN.1 RESET-EN.2 68.33,33.21 v69.47,34.36 | C11.1 91.27,6.04 RESET.1 RESET.2 95.08,1.46 87.63,1.46 86.23,2.86 86.23,11.75 D3.A 84.84,13.15 81.41,13.15 v81.28,13.02 | U2.30 58.99,21.59 59.31,21.27 61.59,21.27 62.1,21.78 62.1,22.8 | 62.1,22.8 62.1,26.35 J3.5 | v63.25,22.8 62.1,22.8
  Bottom 0.254: v72.77,38.42 72.77,37.66 v69.47,34.36 63.63,28.51 J3.5 | v81.28,13.02 80.39,13.02 74.42,18.99 74.42,19.75 73.79,20.39 65.66,20.39 v63.25,22.8
RESET2  (via drill 0.41)
  Top 0.254: U3.24 80.48,42.32 D2.A 82.5,37.4 79.88,37.4 79.38,36.9 79.38,35.37 78.87,34.86 77.34,34.86 76.83,35.37 76.83,37.4 | 76.83,37.4 ICSP1.5 76.83,37.4 | RN5.7 72.26,35.1 v72.26,34.1
  Bottom 0.254: v72.26,34.1 74.3,36.13 74.3,37.4 ICSP1.5
RTS_Y/A
  Top 0.254: J5.2 54.23,51.37 56.64,48.96 56.64,43.63 56.07,43.06 U1.6
RX_A
  Top 0.254: U1.13 49.21,44.33 49.66,44.77 49.66,46.55 49.15,47.06 J5.4
RXL
  Top 0.254: U3.10 69.8,46.02 RX.C
S0RX  (via drill 0.41)
  Top 0.254: RN4.7 72.16,39.04 v71.25,38.17 | U2.2 62.19,9.17 61.76,9.17 60.33,10.61 v60.33,13.53
  Bottom 0.254: v71.25,38.17 71.25,37.4 60.33,26.48 v60.33,13.53
S0TX  (via drill 0.41)
  Top 0.254: RN4.8 72.95,39.51 v74.04,38.42 | v61.21,12.64 61.21,10.48 62.02,9.67 U2.3
  Bottom 0.254: v74.04,38.42 73.53,37.91 73.53,37.15 69.98,33.59 69.09,32.7 | 69.09,32.7 68.96,32.58 | v61.21,12.64 61.21,24.83 62.99,26.61 64.14,26.61 64.9,27.37 64.9,28.51 69.09,32.7
SCK2
  Top 0.254: U3.15 74.82,43.52 74.55,43.25 74.55,41.72 77.6,38.67 ICSP1.3
TWI_SCL  (via drill 0.41)
  Top 0.254: v73.79,4.38 74.06,4.66 RN1.2 | v64.39,7.69 64.39,10.73 v64.9,11.24 | v53.72,19.5 52.49,20.73 U2.43 52.49,23.77 52.07,24.2 R7.2
  Bottom 0.254: J1.4 v64.39,7.69 65.15,8.45 72.39,8.45 74.55,6.29 74.55,5.15 v73.79,4.38 | v64.9,11.24 60.71,11.24 53.72,18.23 v53.72,19.5
TWI_SDA  (via drill 0.41)
  Top 0.254: RN1.1 73.98,5.46 v73.79,5.65 | v65.66,7.69 65.66,9.97 v66.42,10.73 | v52.45,19.5 51.99,19.96 U2.44
  Bottom 0.254: J1.3 66.93,4.64 65.66,5.91 v65.66,7.69 69.98,7.69 71.75,7.69 v73.79,5.65 | v66.42,10.73 66.17,10.48 60.71,10.48 52.45,18.73 v52.45,19.5
TX_Z/B
  Top 0.254: J5.1 56.77,50.87 57.15,50.48 57.15,43.37 56.2,42.42 U1.5
TXL
  Top 0.254: U3.11 71.96,45.52 TX.C
UD+
  Top 0.254: RN2.5 85.66,44.33 86.74,43.25 | 86.74,43.25 87,43.5 87.57,43.5 X2.3 | 86.74,43.25 86.74,39.2 Z2.2
UD-
  Top 0.406: Z1.2 86.76,51.87 87.25,51.37 90.55,48.07 90.55,47.06 89.79,46.29 88.36,46.29 X2.2 85.42,46.73 RN2.8
UGND  (via drill 0.41)
  Top 0.254: U3.28 81.78,44.52 83.44,42.87 C10.2 | v86.74,36.39 86.74,37.66 L1.1
  Top 0.406: C10.2 84.58,42.87 v85.47,41.98 85.47,39.18 85.47,37.91 85.72,37.66 L1.1
  Bottom 0.254: GROUND.1 90.81,36.64 87,36.64 v86.74,36.39
  Bottom 0.406: X2.4 90.55,46.1 90.55,44.26 88.27,41.98 v85.47,41.98
UI_GPIO0
  Top 0.254: U2.15 65.77,15.67 66.67,16.58 JP1.6
UI_GPIO1
  Top 0.254: U2.16 65.38,16.17 67.18,17.97 72.01,17.97 JP1.7
UI_GPIO2
  Top 0.254: U2.17 64.99,16.67 67.44,19.12 JP1.8
UI_GPIO3
  Top 0.254: JP1.5 74.42,17.85 74.42,19.75 73.79,20.39 67.82,20.39 64.6,17.17 U2.18
UI_RXD
  Top 0.254: U2.12 68.19,14.17 69.6,12.77 71.88,12.77 JP1.3
UI_TXD
  Top 0.254: U2.13 68.71,14.67 69.34,14.04 JP1.4
USBVCC
  Top 0.254: U3.31 80.88,46.02 81.41,46.55 81.41,48.07 81.66,48.33 | F1.1 81.03,50.69 81.03,50.36 81.03,50.31 81.03,48.96 81.66,48.33 | C8.1 81.66,48.33
  Top 0.813: F1.1 78.82,53.28 68.33,53.28 64.39,49.34 64.39,34.61 64.39,32.58 65.43,31.54 75.31,31.54 T1.1
USHIELD
  Top 0.406: Z1.1 90.71,53.41 X2.P$2 X2.P$1 90.71,39.18 Z2.1 88.76,37.88 L1.2
UVCC
  Top 0.813: X2.1 87.11,48.13 84.33,50.87 84.37,51.17 F1.2
VIN  (via drill 0.41)
  Top 0.254: v80.9,22.16 80.9,23.05 C2.1 81.66,24.32 v81.66,28.77 | PC1.+ 80.9,17.99 v80.9,19.62 | RN5.6 71.25,35.1 71.25,33.59 71.75,33.09 72.77,33.09 73.28,33.59 77.6,33.59 77.6,33.09 77.85,32.83 80.14,32.83 v80.9,32.07
  Top 0.813: PC1.+ 84.76,16.21 D1.C 85.56,15.81 93.6,15.81 94.87,17.08 94.87,23.69 91.34,27.22 IC1.3
  Bottom 0.254: v80.9,22.16 v80.9,19.62 | v81.66,28.77 81.66,31.31 v80.9,32.07
VUCAP
  Top 0.254: U3.27 81.27,44.02 C10.1
XT1
  Top 0.254: 58.04,29.8 X3.1 59.31,28.53 | U2.33 57.49,25.63 R1.2 58.17,25.72 59.31,26.86 59.31,28.53 | C21.1 60.31,29.53 59.31,28.53
XT2
  Top 0.254: U3.2 79.1,48.6 78.61,49.09 77.6,50.1 | C15.1 69.73,49.58 X1.1 72.88,47.82 74.17,47.82 75.31,48.96 76.45,48.96 77.6,50.1 | 77.6,50.1 R11.2
Z_CTS  (via drill 0.41)
  Top 0.254: v51.18,33.85 51.18,32.58 44.83,26.23 44.83,18.99 45.65,18.17 U2.56 | U1.7 51.37,43.69 v51.18,43.5
  Bottom 0.254: v51.18,43.5 v51.18,33.85
Z_FAST  (via drill 0.41)
  Top 0.254: U1.10 52.65,45.6 v52.07,45.02 | v48.39,33.59 43.31,28.51 43.31,18.23 44.86,16.67 U2.59
  Bottom 0.254: v52.07,45.02 50.8,45.02 48.39,42.61 v48.39,33.59
Z_HDPLX  (via drill 0.41)
  Top 0.254: v47.75,31.69 43.81,27.75 43.81,18.48 45.12,17.17 U2.58 | U1.12 48.83,44.96 49.02,45.15 49.02,46.17 48.64,46.55 v47.88,46.55
  Bottom 0.254: v47.88,46.55 47.24,46.55 45.72,45.02 45.72,33.72 v47.75,31.69
Z_RS485  (via drill 0.41)
  Top 0.254: v47.12,33.59 42.8,29.28 42.8,17.97 44.6,16.17 U2.60 | U1.11 46.8,45.6 46.48,45.28 v46.48,44.64
  Bottom 0.254: v46.48,44.64 46.48,34.23 v47.12,33.59
Z_RTS  (via drill 0.41)
  Top 0.254: v52.07,33.09 52.07,32.45 45.34,25.72 45.34,19.24 45.91,18.67 U2.55 | U1.15 49.47,43.06 50.04,42.48 51.69,42.48 v52.07,42.87
  Bottom 0.254: v52.07,42.87 v52.07,33.09
Z_RX  (via drill 0.41)
  Top 0.254: v54.74,33.47 54.74,32.83 51.05,29.28 51.05,24.32 51.49,23.89 U2.45 51.49,17.03 v52.07,16.45 | RN1.3 74.53,3.86 v73.79,3.11 | U1.8 55.31,44.33 v55.75,43.88
  Bottom 0.254: v55.75,43.88 55.75,34.48 v54.74,33.47 | v73.79,3.11 75.18,4.51 75.18,6.42 72.64,8.96 59.94,8.96 52.45,16.45 v52.07,16.45
Z_TX  (via drill 0.41)
  Top 0.254: v53.47,32.83 50.55,29.91 50.55,24.07 50.99,23.62 U2.46 | U1.16 49.34,42.42 49.78,41.98 v52.96,41.98
  Bottom 0.254: v52.96,41.98 52.96,33.34 v53.47,32.83

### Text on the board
Top: SANDS MOTHERBOARD 002
tSilk: ACT | COMM | ON | POWER | ACT | ALARM | TWI | IDAL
